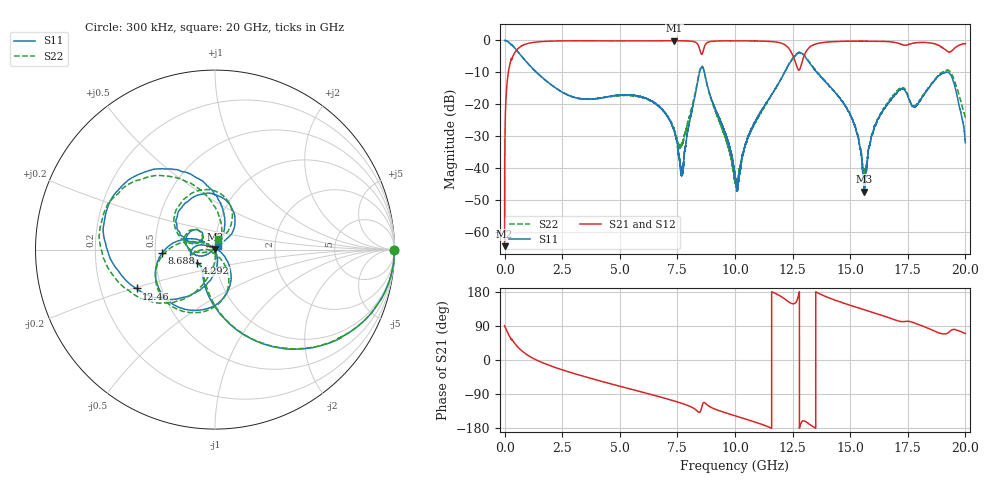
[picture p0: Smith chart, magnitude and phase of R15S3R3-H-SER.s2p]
!{R15S3R3}
!Johanson Technology Inc.
!www.johansontechnology.com
!Test Board Conditions:
!Substrate Type  RO4350B
!Substrate Thickness  20 mil
!Substrate Dk  3.66
!TL Type: GCPW
!TL Trace Width  34 mil
!TL Gap  10 mil
!Electrode orientation  Horizontal
!DUT TOPOLOGY	SERIES
!Mounting Pad LxW  26x52 mil
! Created Sat Feb  6 13:53:59 2021
# hz S ma R 50
! 2 Port Network Data from SP1.SP block
! freq  magS11  angS11  magS21  angS21  magS12  angS12  magS22  angS22
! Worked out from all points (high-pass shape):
!   20001 points, 300 kHz to 20 GHz, reference 50 ohm
!   highest |S21| = -0.09 dB at 7.361 GHz (marker M1); lowest = -64.5 dB at 300 kHz (marker M2)
!   |S21| within 3 dB of the highest: 513.5 MHz to 8.48 GHz (7.967 GHz wide, 177 % of centre); 13.12 GHz to 19.16 GHz (6.042 GHz wide, 37.4 % of centre)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
!   lowest |S11| = -47.4 dB at 15.6 GHz (marker M3), VSWR 1.01, Z = 49.9 + j0.411 ohm
!   |S11| at or under -10 dB: 1.387 GHz to 8.461 GHz (7.074 GHz wide, 144 % of centre); 8.668 GHz to 12.16 GHz (3.488 GHz wide, 33.5 % of centre); 13.55 GHz to 19.13 GHz (5.582 GHz wide, 34.2 % of centre)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
!   |S22| runs from -45.9 to 0.0 dB; largest |S21 - S12| = 0.012
!   S11 on the Smith chart (normalised r, x): 300 kHz: open; 4.292 GHz: 0.81, -0.12; 8.688 GHz: 0.55, -0.02; 12.46 GHz: 0.36, -0.21; 20 GHz: 1.03, +0.04
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300000  1 -0.3  0.0005956 90.9  0.0005994 93.3  0.9979 -0.2
1.243e8  0.9676 -16.2  0.248 73.5  0.2486 73.5  0.9672 -16.1
4.263e8  0.7723 -44.9  0.6305 44.9  0.6322 44.9  0.7721 -44.7
1.3343e9  0.33 -88.8  0.9399 1.4  0.9407 1.3  0.3295 -88.1
3.3343e9  0.1215 -129.8  0.9882 -41.4  0.988 -41.5  0.1219 -132.5
4.2923e9  0.1274 -143.8  0.9851 -57.7  0.9858 -57.7  0.1266 -151.2
6.6673e9  0.09522 165.1  0.9869 -96.1  0.9872 -96.2  0.09491 -176.0
7.3613e9  0.03868 152.2  0.9902 -108.1  0.9896 -108.2  0.04088 179.4
7.7033e9  0.008041 50.3  0.9872 -114.6  0.9873 -114.6  0.0246 -94.1
8.4463e9  0.3007 -87.1  0.7687 -138.3  0.7669 -138.2  0.3146 -89.2
8.6883e9  0.2943 -176.5  0.823 -112.9  0.8231 -112.8  0.2938 -173.9
1.00003e10  0.007262 169.4  0.9865 -147.2  0.9874 -147.2  0.006602 176.0
1.17003e10  0.164 -96.9  0.9517 177.1  0.9523 177.2  0.1634 -105.0
1.24563e10  0.4878 -153.6  0.6407 149.2  0.6467 148.9  0.5007 -147.6
1.28003e10  0.6438 159.9  0.3452 -178.8  0.3488 -179.0  0.6485 168.1
1.33343e10  0.397 101.6  0.8287 -173.8  0.8253 -173.9  0.4077 112.4
1.50163e10  0.06586 59.0  0.9735 144.1  0.9736 144.2  0.06618 63.3
1.56033e10  0.004284 105.9  0.9758 132.6  0.9718 132.9  0.008604 110.4
1.59963e10  0.03755 -148.6  0.9709 125.3  0.9719 125.3  0.03623 -162.5
1.66673e10  0.1048 -162.5  0.9588 111.7  0.9508 111.8  0.1096 -173.8
1.92463e10  0.317 98.4  0.6681 71.6  0.6709 71.9  0.3402 102.0
2e10  0.02485 57.4  0.8903 69.8  0.8873 69.7  0.06336 74.1
